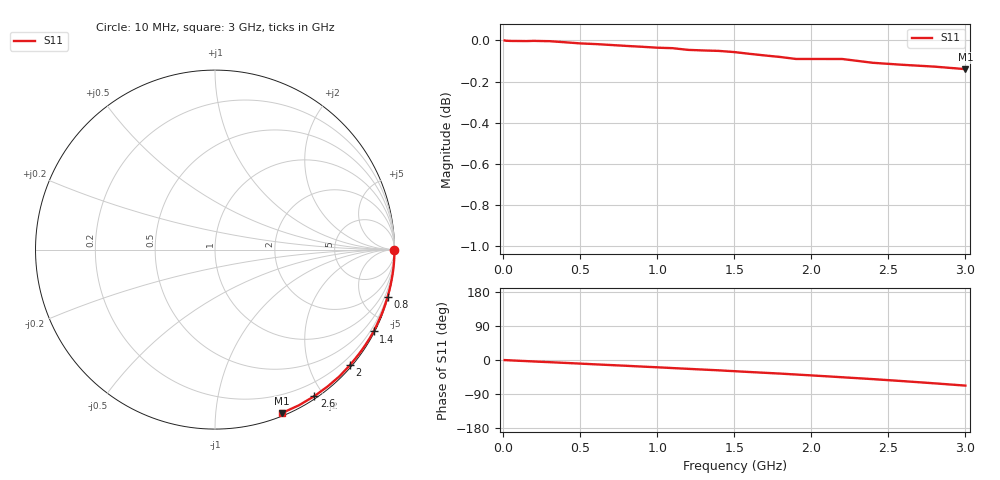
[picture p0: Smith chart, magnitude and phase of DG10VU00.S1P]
! SIEMENS Small Signal Semiconductors
! BAV70
! Silicon Switching Diode in SOT23
! VR = 10 V
! S-Parameters:  May  1995
# GHz  S  MA  R  50
!  f  S11
! GHz  MAG  ANG
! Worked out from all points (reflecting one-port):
!   30 points, 10 MHz to 3 GHz, reference 50 ohm
!   lowest |S11| = -0.1 dB at 3 GHz (marker M1), VSWR 124.55, Z = 1.3 - j74.7 ohm
!   phase of S11 starts at -0 deg and turns -67 deg over the sweep
!   S11 on the Smith chart (normalised r, x): 10 MHz: open; 800 MHz: 0.09, -7.44; 1.4 GHz: 0.05, -4.12; 2 GHz: 0.04, -2.70; 2.6 GHz: 0.03, -1.88; 3 GHz: 0.03, -1.49
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0.01  1 -0.2
0.1  0.9997 -2.0
0.15  0.9996 -2.9
0.2  0.9998 -3.9
0.25  0.9997 -4.8
0.3  0.9996 -5.7
0.4  0.999 -7.6
0.5  0.9983 -9.5
0.6  0.998 -11.5
0.7  0.9975 -13.4
0.8  0.9969 -15.3
0.9  0.9965 -17.3
1  0.996 -19.2
1.1  0.9957 -21.3
1.2  0.9947 -23.3
1.3  0.9944 -25.3
1.4  0.9942 -27.3
1.5  0.9935 -29.5
1.6  0.9925 -31.7
1.7  0.9916 -33.8
1.8  0.9908 -35.9
1.9  0.9897 -38.3
2  0.9897 -40.6
2.2  0.9897 -45.5
2.4  0.9876 -50.5
2.6  0.9864 -55.9
2.8  0.9855 -61.6
3  0.9841 -67.6
